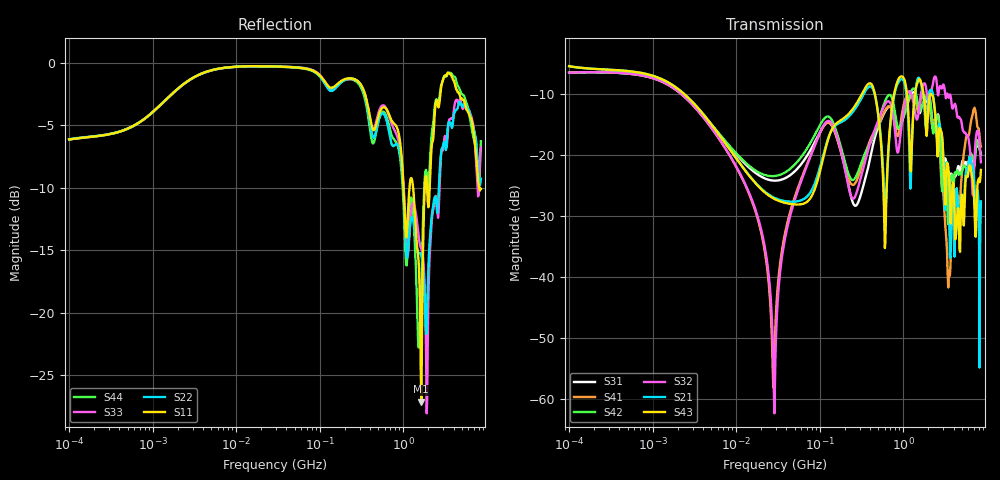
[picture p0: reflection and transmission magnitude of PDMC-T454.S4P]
# Hz S dB R 50
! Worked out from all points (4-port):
!   801 points, 100 kHz to 8.5 GHz, reference 50 ohm
!   strongest paths, dB at 100 kHz, 1.721 MHz, 29.51 MHz, 502.3 MHz, 8.5 GHz:
!     S43: -5.4, -8.4, -27.2, -13.5, -22.4
!     S21: -5.4, -8.4, -27.0, -13.3, -27.6
!     S32: -6.4, -8.8, -53.1, -14.2, -21.1
!     S42: -6.5, -8.8, -23.4, -14.4, -19.9
!     S41: -6.5, -8.9, -47.8, -15.0, -18.6
!     S31: -6.4, -8.8, -24.2, -15.3, -19.7
!   lowest |S11| = -27.1 dB at 1.645 GHz (marker M1), VSWR 1.09, Z = 54.5 + j0.969 ohm
!   |S11| at or under -10 dB: 1.007 GHz to 1.187 GHz (180.4 MHz wide, 16.4 % of centre); 1.312 GHz to 1.81 GHz (497.7 MHz wide, 31.9 % of centre); 8.114 GHz to end of sweep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
100000  -6.14 15.7  -5.37 -14.3  -6.44 -170.3  -6.45 9.7
        -5.36 -14.3  -6.12 15.7  -6.44 9.7  -6.45 -170.3
        -6.44 -170.3  -6.44 9.8  -6.14 15.7  -5.36 -14.3
        -6.45 9.7  -6.45 -170.2  -5.36 -14.3  -6.15 15.6
5443088  -0.55 8.6  -15.49 -65.1  -15.50 107.6  -16.12 -71.0
         -15.49 -65.1  -0.55 8.5  -16.08 -71.0  -15.47 107.5
         -15.51 107.6  -16.08 -71.0  -0.56 8.6  -15.51 -64.9
         -16.12 -71.0  -15.46 107.5  -15.49 -64.9  -0.56 8.5
2.867989e7  -0.30 -1.7  -26.97 -51.4  -24.15 85.6  -52.76 54.8
            -26.97 -51.4  -0.30 -1.9  -62.07 9.6  -23.41 85.2
            -24.15 85.7  -62.34 8.1  -0.30 -1.8  -27.15 -49.5
            -52.81 55.0  -23.40 85.2  -27.15 -49.6  -0.31 -2.3
1.087329e8  -1.29 -13.0  -20.28 -154.7  -15.40 43.8  -15.46 42.9
            -20.27 -154.7  -1.39 -14.6  -15.32 43.8  -14.30 43.8
            -15.40 43.8  -15.32 43.8  -1.27 -14.0  -20.77 -158.3
            -15.45 42.8  -14.29 43.8  -20.77 -158.4  -1.40 -15.2
1.645356e9  -27.13 11.6  -8.46 -14.0  -12.27 -28.2  -10.27 -10.6
            -8.47 -14.0  -15.42 -166.0  -9.58 20.6  -12.06 -35.5
            -12.27 -28.2  -9.58 20.6  -14.89 -179.7  -8.14 -21.1
            -10.27 -10.6  -12.06 -35.4  -8.14 -21.2  -18.42 51.9
3.508736e9  -0.79 -1.7  -25.36 -80.5  -26.78 -65.2  -40.06 5.7
            -25.36 -80.6  -4.76 27.2  -10.56 -52.6  -29.00 -44.0
            -26.75 -65.0  -10.56 -52.5  -4.71 26.8  -22.76 -70.1
            -40.02 5.4  -29.00 -44.1  -22.76 -70.0  -0.86 8.5
8.5e9  -10.09 -6.5  -27.48 54.4  -19.74 -101.0  -18.60 41.6
       -27.57 54.6  -9.28 19.2  -21.12 -76.4  -19.98 -101.0
       -19.74 -100.7  -21.14 -75.7  -6.79 21.9  -22.45 44.5
       -18.56 41.9  -19.91 -100.5  -22.39 44.2  -6.28 -2.7
